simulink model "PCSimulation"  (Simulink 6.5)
settings: Solver=FixedStepDiscrete  SolverMode=SingleTasking  StartTime=0.0  StopTime=inf  FixedStep=samplePeriod  RelTol=1e-3  AbsTol=1e-6
PreLoadFcn:
  | initialize
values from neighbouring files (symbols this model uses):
  actParams = [	bulkModulus   * pressCanon    [Copy of initialize.m]    (also in initialize.m = [bulkModulus	* pressCanon,)
  displFreq = inf    [initialize.m]
  flowCanon = 1.666667e+04    (= 16666.67)    [Copy of initialize.m]    (also in initialize.m)
  forceCanon = 1    [Copy of initialize.m]    (also in initialize.m)
  forceFreq = inf    [initialize.m]
  friction = 5			 				* 0.155000	 				* 0.00444822 				* area1    (= 2.71252900422)    [initialize.m]
  fsamp = 1 / samplePeriod    (= 1024)    [Copy of initialize.m]    (also in initialize.m; rampth.m = 1 / deltaT; randth.m = 1 / deltaT; rspect.m = 1.0 / tsamp)
  gasConstant = 1.8    [Copy of initialize.m]    (also in initialize.m)
  lengthCanon = 1    [Copy of initialize.m]    (also in initialize.m)
  massCanon = 1e-06    [Copy of initialize.m]    (also in initialize.m)
  maxDispl = ( (stroke2 + endLength2) * lengthCanon)'    [Copy of initialize.m]    (also in initialize.m = 576.2)
  maxOilVolume = volume * (1 - (precharge/supplyPress)^(1/gasConstant))    (= 211.391477114)    [Copy of initialize.m]    (also in initialize.m)
  maxVeloc = ( (maxFlow' * flowCanon ./ (area1 * areaCanon)) / velocCanon)'    [Copy of initialize.m]    (also in initialize.m = (maxFlow * flowCanon / (area1 * areaCanon)) / velocCanon; rampth.m = 2 * maxDispl / (nVeloc * deltaT))
  minDispl = (-(stroke1 + endLength1) * lengthCanon)'    [Copy of initialize.m]    (also in initialize.m = -576.2)
  minVeloc = (-(maxFlow' * flowCanon ./ (area2 * areaCanon)) / velocCanon)'    [Copy of initialize.m]    (also in initialize.m = -(maxFlow * flowCanon / (area2 * areaCanon)) / velocCanon)
  nAct = 5    [Copy of initialize.m]    (also in initialize.m = 1)
  nAdcU = 6    [Copy of initialize.m]    (also in initialize.m = 5)
  nDinp = 4    [Copy of initialize.m]    (also in initialize.m)
  nDout = 4    [Copy of initialize.m]    (also in initialize.m)
  nDucU = 2    [Copy of initialize.m]    (also in initialize.m)
  nEncU = 3    [Copy of initialize.m]    (also in initialize.m)
  nUDPInp = 1+6*nAct+nAdcU+nDucU+nEncU+nDout    (= 46)    [Copy of initialize.m]    (also in initialize.m = 10)
  nUDPOut = 1+7*nAct+nAdcU+nDucU+nEncU+nDinp    (= 51)    [Copy of initialize.m]    (also in initialize.m = 12)
  precharge = 3000		 				* 6.894757e-03    (= 20.684271)    [Copy of initialize.m]    (also in initialize.m)
  pumpFlow = 1e20    (= 1e+20)    [Copy of initialize.m]    (also in initialize.m)
  returnPress = 3			 				* 0.1    (= 0.3)    [Copy of initialize.m]    (also in initialize.m)
  samplePeriod = controlPeriod/upsampleFactor    (= 0.0009765625)    [Copy of initialize.m]    (also in initialize.m; viewer.m = eval(getHeaderValue(header, 'DELTA_T')))
  springCanon = 1    [Copy of initialize.m]    (also in initialize.m)
  supplyPress = 280		 				* 0.1    (= 28)    [Copy of initialize.m]    (also in initialize.m)
  upsampleFactor = 1    [Copy of initialize.m]    (also in initialize.m)
  velocCanon = 1    [Copy of initialize.m]    (also in initialize.m)
  volume = 15.15		 				+ (  45		 				    * 2		 				   + 30		 				    * 6 )	 				* 5    (= 1365.15)    [Copy of initialize.m]    (also in initialize.m; quake.m = volume / 231.0)
  volumeCanon = 1e+06    (= 1000000)    [Copy of initialize.m]    (also in initialize.m)
  yieldDispl = 1.0    (= 1)    [initialize.m]
undefined symbols (not defined in the file or in its folder): DiscIntNeverNeededParam, dpforceFreq, mass, spring, staticForce
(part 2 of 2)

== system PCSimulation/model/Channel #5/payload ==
  force : Inport
  Sum : Sum  Inputs=+---
  div : Product  Inputs=*/
  double integrator : S-Function  FunctionName=doubleintegrator  Parameters=maxDispl, minDispl, initDispl, maxVeloc, minVeloc, initVeloc, samplePeriod  mask(Double integrator){maxDispl=maxDispl(id), minDispl=minDispl(id), initDispl=0, maxVeloc=maxVeloc(id)*velocCanon, minVeloc=minVeloc(id)*velocCanon, initVeloc=0, samplePeriod=samplePeriod}
      mask prompts: maxDispl "Maximum displacement"; minDispl "Minimum displacement"; initDispl "Initial displacement"; maxVeloc "Maximum velocity"; minVeloc "Minimum velocity"; initVeloc "Initial velocity"; samplePeriod "Sample period (sec)"
      mask help: Integrates acceleration twice to produce velocity and displacement. When clipping occurs, acceleration, velocity and displacement are adjusted accordingly.
  friction : Subsystem  Orientation=left  mask{friction=friction(id)*forceCanon, yieldDispl=yieldDispl(id)*lengthCanon, hysteresis=0}
      mask prompts: friction "Sliding friction"; yieldDispl "Equiv. yield displacement (in)"; hysteresis "Hysteresis constant"
  mass : Constant  Value=mass(id)*massCanon  OutDataType=sfix(16)  ConRadixGroup=Use specified scaling  OutScaling=2^0  SampleTime=inf  FramePeriod=inf
  spring : Gain  Orientation=left  Gain=spring(id)*springCanon
  static force : Constant  Value=staticForce(id)*forceCanon  OutDataType=sfix(16)  ConRadixGroup=Use specified scaling  OutScaling=2^0  SampleTime=inf  FramePeriod=inf
  term1 : Terminator
  unit dly : UnitDelay  Orientation=left  SampleTime=-1
  veloc units : Gain  Gain=1/velocCanon
  displ : Outport
  veloc : Outport  Port=2
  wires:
  friction/1(force) -> Sum/2  "friction force"
  unit dly/1 -> spring/1
  veloc units/1 -> veloc/1
  Sum/1 -> div/1  "inertial force"
  static force/1 -> Sum/4  "static force"
  force/1 -> Sum/1  "total force"
  mass/1 -> div/2
  spring/1 -> Sum/3  "spring force"
  double integrator/3 -> term1/1
  div/1 -> double integrator/1
  double integrator/1 -> displ/1, unit dly/1
  double integrator/2 -> veloc units/1, friction/1(veloc)

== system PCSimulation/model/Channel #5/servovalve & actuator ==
  note: Auxiliary diagnostic output vector: 1: valve opening 2: C1 pressure 3: C2 pressure 4: delta pressure 5: force 6: velocity 7: C1 flow 8: C2 flow 9: total flow 10: kinematic flow 11: compressibility flow 12: leakage flow 13: C1 oilspring displacement 14: C2 oilspring displacement 15: C1 oilspring velocity 16: C2 oilspring velocity
  note: Note: "1" and "2" denote actuator cylinders on either side of the actuator piston. With positive valve drive, oil is ported into cylinder 1, resulting in positive displacement.
  note: Parameter vector: 1: oil bulk modulus (force/displ^2) 2: servovalve delay (sec) 3: servovalve overlap 4: rated pressure (force/displ^2) 5: rated flow at rated pressure (displ^3/sec) 6: nominal flow at rated pressure (displ^3/sec) 7: actuator piston area 1 (displ^2) 8: actuator piston area 2 (displ^2) 9: actuator usable stroke 1 (displ) 10: actuator usable stroke 2 (displ) 11: actuator end cushion length 1 (displ) 12: actuator end cushion length 2 (displ) 13: additional port volume 1 (displ^3) 14: additional port volume 1 (displ^3) 15: actuator parasitic damping factor 16: cross-chamber leakage factor (flow/press) 17: ratio port openings according to area 18: sample period (sec) Conversion factors used for converting signals from external (user) to internal (canonical) units: 19: displacement 20: velocity 21: force 22: pressure 23: flow
  cmd : Inport
  displ : Inport  Port=2
  veloc : Inport  Port=3
  spl press : Inport  Port=4
  rtn press : Inport  Port=5
  abs : Abs  SaturateOnIntegerOverflow=on  SampleTime=-1
  actuator : S-Function  FunctionName=Actuator  Parameters=params
  total flow sel : Selector  InputType=Vector  ElementSrc=Internal  Elements=9  RowSrc=Internal  Rows=1  ColumnSrc=Internal  Columns=1  IndexIsStartValue=off
  force : Outport
  flow : Outport  Port=2
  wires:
  abs/1 -> flow/1
  total flow sel/1 -> abs/1
  actuator/2 -> total flow sel/1
  veloc/1 -> actuator/3
  displ/1 -> actuator/2
  actuator/1 -> force/1
  cmd/1 -> actuator/1
  rtn press/1 -> actuator/5
  spl press/1 -> actuator/4

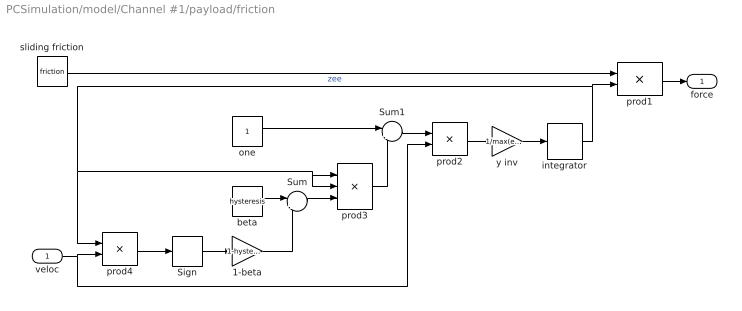
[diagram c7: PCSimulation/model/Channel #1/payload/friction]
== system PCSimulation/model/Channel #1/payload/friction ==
  veloc : Inport
  1-beta : Gain  Gain=1-hysteresis
  Sign : Signum
  Sum : Sum  Inputs=|++
  Sum1 : Sum  Inputs=|+-
  beta : Constant  Value=hysteresis  OutDataType=sfix(16)  ConRadixGroup=Use specified scaling  OutScaling=2^0  SampleTime=inf  FramePeriod=inf
  integrator : DiscreteIntegrator  SampleTime=-1  LimitOutput=on  UpperSaturationLimit=1  LowerSaturationLimit=-1  ICPrevOutput=DiscIntNeverNeededParam  ICPrevScaledInput=DiscIntNeverNeededParam
  one : Constant  Value=1  OutDataType=sfix(16)  ConRadixGroup=Use specified scaling  OutScaling=2^0  SampleTime=inf  FramePeriod=inf
  prod1 : Product
  prod2 : Product
  prod3 : Product  Inputs=3
  prod4 : Product
  sliding friction : Constant  Value=friction  OutDataType=sfix(16)  ConRadixGroup=Use specified scaling  OutScaling=2^0  SampleTime=inf  FramePeriod=inf
  y inv : Gain  Gain=1/max(eps, yieldDispl)
  force : Outport
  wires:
  sliding friction/1 -> prod1/1
  prod1/1 -> force/1
  veloc/1 -> prod4/2, prod2/2
  prod4/1 -> Sign/1
  Sign/1 -> 1-beta/1
  1-beta/1 -> Sum/2
  beta/1 -> Sum/1
  Sum/1 -> prod3/3
  one/1 -> Sum1/1
  prod3/1 -> Sum1/2
  Sum1/1 -> prod2/1
  prod2/1 -> y inv/1
  y inv/1 -> integrator/1
  integrator/1 -> prod1/2, prod4/1, prod3/1, prod3/2  "zee"

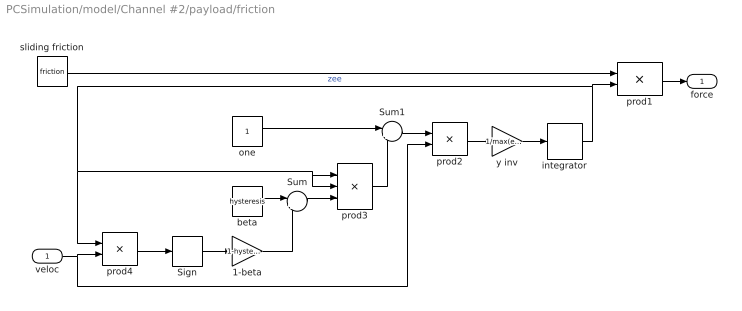
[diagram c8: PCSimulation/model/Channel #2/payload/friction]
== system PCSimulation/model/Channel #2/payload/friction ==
  veloc : Inport
  1-beta : Gain  Gain=1-hysteresis
  Sign : Signum
  Sum : Sum  Inputs=|++
  Sum1 : Sum  Inputs=|+-
  beta : Constant  Value=hysteresis  OutDataType=sfix(16)  ConRadixGroup=Use specified scaling  OutScaling=2^0  SampleTime=inf  FramePeriod=inf
  integrator : DiscreteIntegrator  SampleTime=-1  LimitOutput=on  UpperSaturationLimit=1  LowerSaturationLimit=-1  ICPrevOutput=DiscIntNeverNeededParam  ICPrevScaledInput=DiscIntNeverNeededParam
  one : Constant  Value=1  OutDataType=sfix(16)  ConRadixGroup=Use specified scaling  OutScaling=2^0  SampleTime=inf  FramePeriod=inf
  prod1 : Product
  prod2 : Product
  prod3 : Product  Inputs=3
  prod4 : Product
  sliding friction : Constant  Value=friction  OutDataType=sfix(16)  ConRadixGroup=Use specified scaling  OutScaling=2^0  SampleTime=inf  FramePeriod=inf
  y inv : Gain  Gain=1/max(eps, yieldDispl)
  force : Outport
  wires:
  integrator/1 -> prod3/2, prod3/1, prod4/1, prod1/2  "zee"
  y inv/1 -> integrator/1
  prod2/1 -> y inv/1
  Sum1/1 -> prod2/1
  prod3/1 -> Sum1/2
  one/1 -> Sum1/1
  Sum/1 -> prod3/3
  beta/1 -> Sum/1
  1-beta/1 -> Sum/2
  Sign/1 -> 1-beta/1
  prod4/1 -> Sign/1
  veloc/1 -> prod2/2, prod4/2
  prod1/1 -> force/1
  sliding friction/1 -> prod1/1

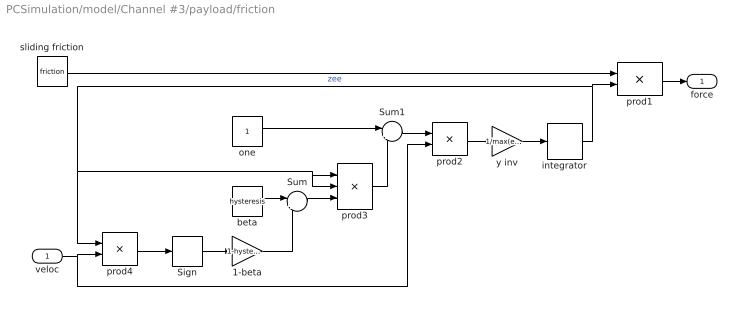
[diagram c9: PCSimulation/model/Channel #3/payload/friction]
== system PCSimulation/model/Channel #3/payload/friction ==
  veloc : Inport
  1-beta : Gain  Gain=1-hysteresis
  Sign : Signum
  Sum : Sum  Inputs=|++
  Sum1 : Sum  Inputs=|+-
  beta : Constant  Value=hysteresis  OutDataType=sfix(16)  ConRadixGroup=Use specified scaling  OutScaling=2^0  SampleTime=inf  FramePeriod=inf
  integrator : DiscreteIntegrator  SampleTime=-1  LimitOutput=on  UpperSaturationLimit=1  LowerSaturationLimit=-1  ICPrevOutput=DiscIntNeverNeededParam  ICPrevScaledInput=DiscIntNeverNeededParam
  one : Constant  Value=1  OutDataType=sfix(16)  ConRadixGroup=Use specified scaling  OutScaling=2^0  SampleTime=inf  FramePeriod=inf
  prod1 : Product
  prod2 : Product
  prod3 : Product  Inputs=3
  prod4 : Product
  sliding friction : Constant  Value=friction  OutDataType=sfix(16)  ConRadixGroup=Use specified scaling  OutScaling=2^0  SampleTime=inf  FramePeriod=inf
  y inv : Gain  Gain=1/max(eps, yieldDispl)
  force : Outport
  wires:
  sliding friction/1 -> prod1/1
  prod1/1 -> force/1
  veloc/1 -> prod4/2, prod2/2
  prod4/1 -> Sign/1
  Sign/1 -> 1-beta/1
  1-beta/1 -> Sum/2
  beta/1 -> Sum/1
  Sum/1 -> prod3/3
  one/1 -> Sum1/1
  prod3/1 -> Sum1/2
  Sum1/1 -> prod2/1
  prod2/1 -> y inv/1
  y inv/1 -> integrator/1
  integrator/1 -> prod1/2, prod4/1, prod3/1, prod3/2  "zee"

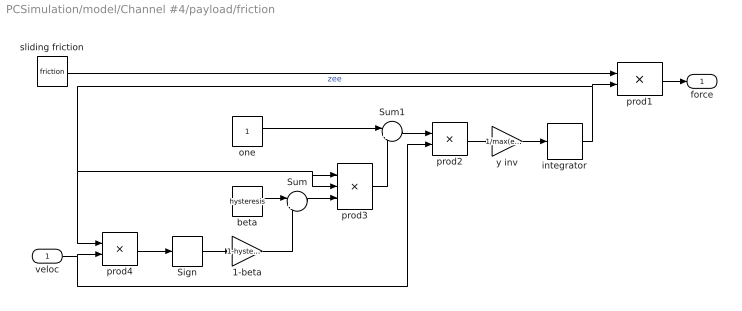
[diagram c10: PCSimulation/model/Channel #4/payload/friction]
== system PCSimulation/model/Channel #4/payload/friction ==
  veloc : Inport
  1-beta : Gain  Gain=1-hysteresis
  Sign : Signum
  Sum : Sum  Inputs=|++
  Sum1 : Sum  Inputs=|+-
  beta : Constant  Value=hysteresis  OutDataType=sfix(16)  ConRadixGroup=Use specified scaling  OutScaling=2^0  SampleTime=inf  FramePeriod=inf
  integrator : DiscreteIntegrator  SampleTime=-1  LimitOutput=on  UpperSaturationLimit=1  LowerSaturationLimit=-1  ICPrevOutput=DiscIntNeverNeededParam  ICPrevScaledInput=DiscIntNeverNeededParam
  one : Constant  Value=1  OutDataType=sfix(16)  ConRadixGroup=Use specified scaling  OutScaling=2^0  SampleTime=inf  FramePeriod=inf
  prod1 : Product
  prod2 : Product
  prod3 : Product  Inputs=3
  prod4 : Product
  sliding friction : Constant  Value=friction  OutDataType=sfix(16)  ConRadixGroup=Use specified scaling  OutScaling=2^0  SampleTime=inf  FramePeriod=inf
  y inv : Gain  Gain=1/max(eps, yieldDispl)
  force : Outport
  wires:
  integrator/1 -> prod3/2, prod3/1, prod4/1, prod1/2  "zee"
  y inv/1 -> integrator/1
  prod2/1 -> y inv/1
  Sum1/1 -> prod2/1
  prod3/1 -> Sum1/2
  one/1 -> Sum1/1
  Sum/1 -> prod3/3
  beta/1 -> Sum/1
  1-beta/1 -> Sum/2
  Sign/1 -> 1-beta/1
  prod4/1 -> Sign/1
  veloc/1 -> prod2/2, prod4/2
  prod1/1 -> force/1
  sliding friction/1 -> prod1/1

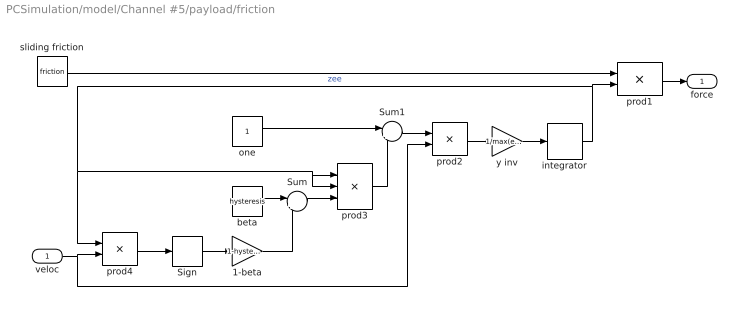
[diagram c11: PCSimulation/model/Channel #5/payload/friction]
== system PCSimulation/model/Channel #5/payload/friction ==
  veloc : Inport
  1-beta : Gain  Gain=1-hysteresis
  Sign : Signum
  Sum : Sum  Inputs=|++
  Sum1 : Sum  Inputs=|+-
  beta : Constant  Value=hysteresis  OutDataType=sfix(16)  ConRadixGroup=Use specified scaling  OutScaling=2^0  SampleTime=inf  FramePeriod=inf
  integrator : DiscreteIntegrator  SampleTime=-1  LimitOutput=on  UpperSaturationLimit=1  LowerSaturationLimit=-1  ICPrevOutput=DiscIntNeverNeededParam  ICPrevScaledInput=DiscIntNeverNeededParam
  one : Constant  Value=1  OutDataType=sfix(16)  ConRadixGroup=Use specified scaling  OutScaling=2^0  SampleTime=inf  FramePeriod=inf
  prod1 : Product
  prod2 : Product
  prod3 : Product  Inputs=3
  prod4 : Product
  sliding friction : Constant  Value=friction  OutDataType=sfix(16)  ConRadixGroup=Use specified scaling  OutScaling=2^0  SampleTime=inf  FramePeriod=inf
  y inv : Gain  Gain=1/max(eps, yieldDispl)
  force : Outport
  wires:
  sliding friction/1 -> prod1/1
  prod1/1 -> force/1
  veloc/1 -> prod4/2, prod2/2
  prod4/1 -> Sign/1
  Sign/1 -> 1-beta/1
  1-beta/1 -> Sum/2
  beta/1 -> Sum/1
  Sum/1 -> prod3/3
  one/1 -> Sum1/1
  prod3/1 -> Sum1/2
  Sum1/1 -> prod2/1
  prod2/1 -> y inv/1
  y inv/1 -> integrator/1
  integrator/1 -> prod1/2, prod4/1, prod3/1, prod3/2  "zee"
